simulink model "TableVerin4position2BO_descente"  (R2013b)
settings: Solver=ode15s  StartTime=0.0  StopTime=2  RelTol=1e-3
undefined symbols (not defined in the file): deg, kg, m, mm, N, rad, s, X, Y, Z
libraries: sm_lib x907, fl_lib x25, nesl_utility x19, elec_lib x3, sdl_lib x2
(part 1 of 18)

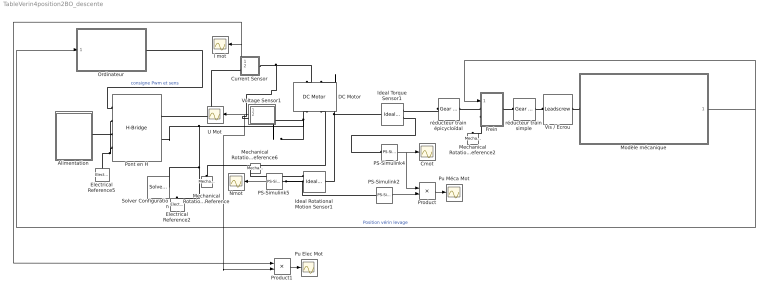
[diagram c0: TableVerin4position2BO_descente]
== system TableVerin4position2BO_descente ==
  Alimentation : Subsystem
  Cmot : Scope
  Current Sensor : Subsystem
  DC Motor : elec_lib/Actuators & Drivers/Rotational Actuators/DC Motor  parameterization=1  Ra=0.53333333 Ohm  La=1600e-6 H  emf_or_torque=2  Kv=0.0637 V/rpm  Ki=0.05555555 N*m/A  T_stall=3e-3*4000/(2*pi*6.25) N*m  w_max=3250 rpm  w_rated=2375 rpm  P_rated=19 W  V_rated=24 V  J=32e-5 kg*m^2  lam_param=2  lam=1e-08 N*m/(rad/s)  i_noload=1.1 A  V_i_noload=24 V  speed0=0 rpm  current_Log=off  voltage_Log=off  power_Log=off  i2r_Log=off  torque_Log=off  speed_Log=off  LocalVarNames=|current|voltage|power|i2r|torque|speed  LocalVarDescs=|Current (A)|Voltage (V)|Power (W)|Electrical losses (W)|Torque (Nm)|Angular speed (rad/s)  LocalVarLogging=[0 0 0 0 0 0]  alpha=0.00393 1/K  Tmeas=25 C  thermal_mass=100 J/K  initial_temperature=25 C
  Electrical Reference2 : fl_lib/Electrical/Electrical Elements/Electrical Reference  i_Log=off  LocalVarNames=|i  LocalVarDescs=|i  LocalVarLogging=[]
  Electrical Reference5 : fl_lib/Electrical/Electrical Elements/Electrical Reference  i_Log=off  LocalVarNames=|i  LocalVarDescs=|i  LocalVarLogging=[]
  Frein : Subsystem
  I mot : Scope
  Ideal Rotational Motion Sensor1 : fl_lib/Mechanical/Mechanical Sensors/Ideal Rotational Motion Sensor  offset=0 deg  w_Log=off  t_Log=off  phi_Log=off  LocalVarNames=|w|t|phi  LocalVarDescs=|w|t|phi  LocalVarLogging=[]
  Ideal Torque Sensor1 : fl_lib/Mechanical/Mechanical Sensors/Ideal Torque Sensor  w_Log=off  t_Log=off  LocalVarNames=|w|t  LocalVarDescs=|w|t  LocalVarLogging=[0 0]
  Mechanical Rotational Reference : fl_lib/Mechanical/Rotational Elements/Mechanical Rotational Reference  t_Log=off  LocalVarNames=|t  LocalVarDescs=|t  LocalVarLogging=[]
  Mechanical Rotational Reference2 : fl_lib/Mechanical/Rotational Elements/Mechanical Rotational Reference  t_Log=off  LocalVarNames=|t  LocalVarDescs=|t  LocalVarLogging=[]
  Mechanical Rotational Reference6 : fl_lib/Mechanical/Rotational Elements/Mechanical Rotational Reference  t_Log=off  LocalVarNames=|t  LocalVarDescs=|t  LocalVarLogging=[]
  Modèle mécanique : Subsystem
  Nmot : Scope
  Ordinateur : Subsystem
  PS-Simulink2 : nesl_utility/PS-Simulink Converter  PhysicalDomain=network_engine_domain  SubClassName=ps_output  LeftPortType=input  RightPortType=output  PseudoPeriodic=off  Frequencies=[]  Unit=rad/s  AffineConversion=off
  PS-Simulink4 : nesl_utility/PS-Simulink Converter  PhysicalDomain=network_engine_domain  SubClassName=ps_output  LeftPortType=input  RightPortType=output  PseudoPeriodic=off  Frequencies=[]  Unit=N*m  AffineConversion=off
  PS-Simulink5 : nesl_utility/PS-Simulink Converter  PhysicalDomain=network_engine_domain  SubClassName=ps_output  LeftPortType=input  RightPortType=output  PseudoPeriodic=off  Frequencies=[]  Unit=rpm  AffineConversion=off
  Pont en H : elec_lib/Actuators & Drivers/Drivers/H-Bridge  Venable=2.5 V  Vmax=5 V  Vreverse=2.5 V  Vbrake=2.5 V  Vm=24 V  pwm_or_av=2  discontinuous=0  freewheeling_mode=1  freewheeling_mode_disc=1  Ron=0.1 Ohm  Don=0.1 Ohm  Rload=10 Ohm  Lload=1e-5 H  F=10 kHz  w_vec=[1, 2] s  i_vec=[1, 2] A  vMatrix=[1, 2; 3, 4] V  iENA_Log=off  iREV_Log=off  iBRK_Log=off  i2_Log=off  v_lag_Log=off  LocalVarNames=|current|voltage|power  LocalVarDescs=|Load current (A)|Load voltage (V)|Load power (W)  LocalVarLogging=[0 0 0]
  Product : Product
  Product1 : Product
  Pu Elec Mot : Scope
  Pu Méca Mot : Scope
  Solver Configuration : nesl_utility/Solver Configuration  PhysicalDomain=network_engine_domain  SubClassName=solver  LeftPortType=input  RightPortType=generic  Accelerate=off  Tones=[]  Harmonics=[]  SimulateNoise=off  Profile=off  UseLocalSampling=off  EnableSwitchedLinearOptims=on  FrequencyDomain=off  UseCCode=off  RelTol=0.001  AbsTol=1e-06  MinStep=1e-09  ToWorkspace=off  DoDC=off  ResidualTolerance=1e-09  UseLocalSolver=off  LocalSolverChoice=NE_BACKWARD_EULER_ADVANCER  LocalSolverSampleTime=0.001  DoFixedCost=off  MaxNonlinIter=3  MaxModeIter=2  LinearAlgebra=Sparse  DelaysMemoryBudget=1024
  U Mot : Scope
  Vis / Ecrou : sdl_lib/Gears/Rotational- Translational/Leadscrew  Lead=0.008 m  helix_type=1  friction_model=2  friction_parameterization=1  lambda=13 deg  alpha=14.5 deg  fr_coeff=0.08  eff_sn=0.75  eff_ns=0.45  mu_visc=0 N*m/(rad/s)  v_thr=0.001 m/s  LocalVarLogging=[]
  Voltage Sensor1 : Subsystem
  réducteur train simple : fl_lib/Mechanical/Mechanisms/Gear Box  ratio=2.98  t_in_Log=off  t_out_Log=off  LocalVarNames=|torque_inp|ang_velocity_inp|power  LocalVarDescs=|Input shaft torque (N*m)|Input shaft angular velocity (rad/s)|Power transmitted by the box (W)  LocalVarLogging=[0 0 0]
  réducteur train épicycloïdal : fl_lib/Mechanical/Mechanisms/Gear Box  ratio=15.44  t_in_Log=off  t_out_Log=off  LocalVarNames=|torque_inp|ang_velocity_inp|power  LocalVarDescs=|Input shaft torque (N*m)|Input shaft angular velocity (rad/s)|Power transmitted by the box (W)  LocalVarLogging=[0 0 0]
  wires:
  Modèle mécanique/1(position) -> Frein/1(freinage), Ordinateur/1(In1)  "Position vérin levage"
  PS-Simulink5/1 -> Nmot/1
  PS-Simulink4/1 -> Product/1, Cmot/1
  Product/1 -> Pu Méca Mot/1
  PS-Simulink2/1 -> Product/2
  Current Sensor/1(i) -> I mot/1, Product1/1
  Product1/1 -> Pu Elec Mot/1
  Voltage Sensor1/2(VuMot2) -> U Mot/1, Product1/2
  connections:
  Vis / Ecrou/LConn1 -- réducteur train simple/RConn1
  Mechanical Rotational Reference/LConn1 -- DC Motor/RConn2
  Frein/LConn2 -- Mechanical Rotational Reference2/LConn1
  Frein/RConn1 -- réducteur train simple/LConn1
  Vis / Ecrou/RConn1 -- Modèle mécanique/LConn1
  DC Motor/RConn1 -- Electrical Reference2/LConn1 -- Solver Configuration/RConn1 -- Pont en H/RConn2 -- Voltage Sensor1/LConn1
  Pont en H/LConn2 -- Electrical Reference5/LConn1 -- Pont en H/LConn4
  Pont en H/LConn1 -- Ordinateur/RConn1  "consigne Pwm et sens"
  Alimentation/RConn1 -- Pont en H/LConn3
  Frein/LConn1 -- réducteur train épicycloïdal/RConn1
  Ideal Rotational Motion Sensor1/LConn1 -- Ideal Torque Sensor1/LConn1 -- DC Motor/LConn2
  Voltage Sensor1/RConn1 -- DC Motor/LConn1 -- Current Sensor/LConn1
  Current Sensor/RConn1 -- Pont en H/RConn1
  Mechanical Rotational Reference6/LConn1 -- Ideal Rotational Motion Sensor1/RConn1
  PS-Simulink5/LConn1 -- PS-Simulink2/LConn1 -- Ideal Rotational Motion Sensor1/RConn2
  Ideal Torque Sensor1/RConn2 -- PS-Simulink4/LConn1
  réducteur train épicycloïdal/LConn1 -- Ideal Torque Sensor1/RConn1

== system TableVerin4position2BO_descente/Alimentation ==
  Constant3 : Constant  Value=5
  Controlled Voltage Source1 : fl_lib/Electrical/Electrical Sources/Controlled Voltage Source  i_Log=off  v_Log=off  LocalVarNames=|i|v  LocalVarDescs=|i|v  LocalVarLogging=[0 0]
  Electrical Reference4 : fl_lib/Electrical/Electrical Elements/Electrical Reference  i_Log=off  LocalVarNames=|i  LocalVarDescs=|i  LocalVarLogging=[]
  Simulink-PS Converter1 : nesl_utility/Simulink-PS Converter  PhysicalDomain=network_engine_domain  SubClassName=ps_input  LeftPortType=input  RightPortType=output  PseudoPeriodic=off  Frequencies=[]  NoiseDistribution=none  NoiseParameters=[]  Unit=V  AffineConversion=off  InputFiltering=off  SimscapeFilterOrder=1  InputFilterTimeConstant=0.001  UdotUserProvided=1
  Conn1 : PMIOPort  Port=1  Side=Right
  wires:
  Constant3/1 -> Simulink-PS Converter1/1
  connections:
  Electrical Reference4/LConn1 -- Controlled Voltage Source1/RConn2
  Simulink-PS Converter1/RConn1 -- Controlled Voltage Source1/RConn1
  Controlled Voltage Source1/LConn1 -- Conn1/RConn1

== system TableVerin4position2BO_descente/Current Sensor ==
  Current Sensor : fl_lib/Electrical/Electrical Sensors/Current Sensor  i1_Log=off  v1_Log=off  LocalVarNames=|i1|v1  LocalVarDescs=|i1|v1  LocalVarLogging=[]
  PS-Simulink Converter 2 : nesl_utility/PS-Simulink Converter  PhysicalDomain=network_engine_domain  SubClassName=ps_output  LeftPortType=input  RightPortType=output  PseudoPeriodic=off  Frequencies=[]  Unit=A  AffineConversion=off
  Volts per unit current : Gain
  + : PMIOPort  Port=1  Side=Right
  - : PMIOPort  Port=2  Side=Left
  i : Outport
  V_i : Outport  Port=2
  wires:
  PS-Simulink Converter 2/1 -> Volts per unit current/1, i/1  "Current (A)"
  Volts per unit current/1 -> V_i/1  "Volts"
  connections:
  +/RConn1 -- Current Sensor/LConn1
  -/RConn1 -- Current Sensor/RConn2
  Current Sensor/RConn1 -- PS-Simulink Converter 2/LConn1

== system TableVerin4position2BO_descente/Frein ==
  note: 240 ou 0
  freinage : Inport
  Constant1 : Constant  Value=0
  Constant2 : Constant  Value=240
  Couple1 : Scope
  Couple2 : Scope
  Ideal Rotational Motion Sensor1 : fl_lib/Mechanical/Mechanical Sensors/Ideal Rotational Motion Sensor  offset=0 deg  w_Log=off  t_Log=off  phi_Log=off  LocalVarNames=|w|t|phi  LocalVarDescs=|w|t|phi  LocalVarLogging=[]
  Ideal Torque Sensor1 : fl_lib/Mechanical/Mechanical Sensors/Ideal Torque Sensor  w_Log=off  t_Log=off  LocalVarNames=|w|t  LocalVarDescs=|w|t  LocalVarLogging=[0 0]
  Ideal Torque Sensor2 : fl_lib/Mechanical/Mechanical Sensors/Ideal Torque Sensor  w_Log=off  t_Log=off  LocalVarNames=|w|t  LocalVarDescs=|w|t  LocalVarLogging=[0 0]
  Loaded-Contact Rotational Friction : sdl_lib/Brakes & Detents/Rotational/Loaded-Contact Rotational Friction  geometry_model=1  r_eff=50 mm  d_o=150 mm  d_i=100 mm  friction_model=1  mu_coulomb=0.2  mu_w_vector=[ 0 0.1 0.2 0.3 0.4 0.5 1 2 5 10 100 1000 ] rad/s  mu_coulomb_vector=[ 0.29 0.28 0.26 0.22 0.21 0.2 0.2 0.19 0.19 0.19 0.19 0.19 ]  mu_interp_method=1  mu_extrap_method=1  mu_static=0.21  w_tol=0.001 rad/s  force_min=0.01 N  mu_visc=0 N*m/(rad/s)  initial_state_locked=0  LocalVarLogging=[]
  Mechanical Rotational Reference6 : fl_lib/Mechanical/Rotational Elements/Mechanical Rotational Reference  t_Log=off  LocalVarNames=|t  LocalVarDescs=|t  LocalVarLogging=[]
  N1 : Scope
  PS-Simulink1 : nesl_utility/PS-Simulink Converter  PhysicalDomain=network_engine_domain  SubClassName=ps_output  LeftPortType=input  RightPortType=output  PseudoPeriodic=off  Frequencies=[]  Unit=N*m  AffineConversion=off
  PS-Simulink4 : nesl_utility/PS-Simulink Converter  PhysicalDomain=network_engine_domain  SubClassName=ps_output  LeftPortType=input  RightPortType=output  PseudoPeriodic=off  Frequencies=[]  Unit=N*m  AffineConversion=off
  PS-Simulink5 : nesl_utility/PS-Simulink Converter  PhysicalDomain=network_engine_domain  SubClassName=ps_output  LeftPortType=input  RightPortType=output  PseudoPeriodic=off  Frequencies=[]  Unit=rpm  AffineConversion=off
  Simulink-PS Converter : nesl_utility/Simulink-PS Converter  PhysicalDomain=network_engine_domain  SubClassName=ps_input  LeftPortType=input  RightPortType=output  PseudoPeriodic=off  Frequencies=[]  NoiseDistribution=none  NoiseParameters=[]  Unit=N  AffineConversion=off  InputFiltering=off  SimscapeFilterOrder=1  InputFilterTimeConstant=0.001  UdotUserProvided=1
  Switch1 : Switch  Criteria=u2 > Threshold  Threshold=-10.172
  force : Scope
  out : PMIOPort  Port=1  Side=Right
  In : PMIOPort  Port=2  Side=Left
  bâti : PMIOPort  Port=3  Side=Left
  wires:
  Switch1/1 -> force/1, Simulink-PS Converter/1
  PS-Simulink5/1 -> N1/1
  PS-Simulink4/1 -> Couple1/1
  Constant1/1 -> Switch1/1
  Constant2/1 -> Switch1/3
  freinage/1 -> Switch1/2
  PS-Simulink1/1 -> Couple2/1
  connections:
  Loaded-Contact Rotational Friction/RConn1 -- Ideal Torque Sensor1/RConn1 -- Ideal Torque Sensor2/LConn1
  PS-Simulink5/LConn1 -- Ideal Rotational Motion Sensor1/RConn2
  Ideal Torque Sensor1/RConn2 -- PS-Simulink4/LConn1
  Loaded-Contact Rotational Friction/LConn1 -- Simulink-PS Converter/RConn1
  Mechanical Rotational Reference6/LConn1 -- Ideal Rotational Motion Sensor1/RConn1
  Ideal Rotational Motion Sensor1/LConn1 -- Ideal Torque Sensor1/LConn1 -- In/RConn1
  bâti/RConn1 -- Loaded-Contact Rotational Friction/LConn2
  Ideal Torque Sensor2/RConn2 -- PS-Simulink1/LConn1
  Ideal Torque Sensor2/RConn1 -- out/RConn1

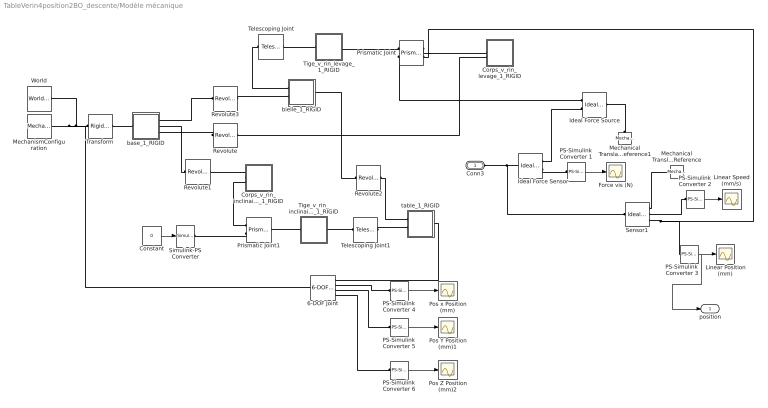
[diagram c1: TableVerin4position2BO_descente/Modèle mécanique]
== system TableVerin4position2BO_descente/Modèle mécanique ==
  6-DOF Joint : sm_lib/Joints/6-DOF Joint  SenseConstraintForceX=off  SenseConstraintForceY=off  SenseConstraintForceZ=off  SenseConstraintTorqueX=off  SenseConstraintTorqueY=off  SenseConstraintTorqueZ=off  ConstraintWrenchDir=FollowerOnBase  ConstraintWrenchFrame=BaseFrame  PxEquilibriumPosition=0  PxEquilibriumPositionUnits=m  PxSpringStiffness=0  PxSpringStiffnessUnits=N/m  PxDampingCoefficient=0  PxDampingCoefficientUnits=N/(m/s)  PxTorqueActuationMode=NoTorque  PxMotionActuationMode=ComputedMotion  PxSensePosition=on  PxSenseVelocity=off  PxSenseAcceleration=off  PxSenseTorqueForce=off  PxPositionTargetValue=0  PxPositionTargetValueUnits=m  PxPositionTargetSpecify=off  PxPositionTargetPriority=High  PxVelocityTargetValue=0  PxVelocityTargetValueUnits=m/s  PxVelocityTargetSpecify=off  PxVelocityTargetPriority=High  PyEquilibriumPosition=0  PyEquilibriumPositionUnits=m  PySpringStiffness=0  PySpringStiffnessUnits=N/m  PyDampingCoefficient=0  PyDampingCoefficientUnits=N/(m/s)  PyTorqueActuationMode=NoTorque  PyMotionActuationMode=ComputedMotion  PySensePosition=on  PySenseVelocity=off  PySenseAcceleration=off  PySenseTorqueForce=off  PyPositionTargetValue=0  PyPositionTargetValueUnits=m  PyPositionTargetSpecify=off  PyPositionTargetPriority=High  PyVelocityTargetValue=0  PyVelocityTargetValueUnits=m/s  PyVelocityTargetSpecify=off  PyVelocityTargetPriority=High  PzEquilibriumPosition=0  PzEquilibriumPositionUnits=m  PzSpringStiffness=0  PzSpringStiffnessUnits=N/m  PzDampingCoefficient=0  PzDampingCoefficientUnits=N/(m/s)  PzTorqueActuationMode=NoTorque  PzMotionActuationMode=ComputedMotion  PzSensePosition=on  PzSenseVelocity=off  PzSenseAcceleration=off  PzSenseTorqueForce=off  PzPositionTargetValue=0  PzPositionTargetValueUnits=m  PzPositionTargetSpecify=off  PzPositionTargetPriority=High  PzVelocityTargetValue=0  PzVelocityTargetValueUnits=m/s  PzVelocityTargetSpecify=off  PzVelocityTargetPriority=High  SphDefPosRotationMethod=None  SphDefPosRotationAngleUnits=deg  SphDefPosRotationStandardAxis=+Z  SphDefPosRotationAngle=0  SphDefPosRotationArbitraryAxis=[0 0 1]  SphDefPosFollAlignAxisA=+X  SphDefPosBaseAlignAxisA=+Y  SphDefPosFollAlignAxisB=+Y  SphDefPosBaseAlignAxisB=+Z  SphEqPosRotationMethod=None  SphEqPosRotationAngleUnits=deg  SphEqPosRotationStandardAxis=+Z  SphEqPosRotationAngle=0  SphEqPosRotationArbitraryAxis=[0 0 1]  SphEqPosFollAlignAxisA=+X  SphEqPosBaseAlignAxisA=+Y  SphEqPosFollAlignAxisB=+Y  SphEqPosBaseAlignAxisB=+Z  SphSpringStiffness=0  SphSpringStiffnessUnits=N*m/deg  SphDampingCoefficient=0  SphDampingCoefficientUnits=N*m/(deg/s)  SphActuateTorqueX=off  SphActuateTorqueY=off  SphActuateTorqueZ=off  SphActuateTorque=off  SphTorqueActuationMode=NoTorque  SphMotionActuationMode=ComputedMotion  SphActuationFrame=BaseFrame  SphSensePosition=off  SphSenseVelocityX=off  SphSenseVelocityY=off  SphSenseVelocityZ=off  SphSenseVelocity=off  SphSenseAccelerationX=off  SphSenseAccelerationY=off  SphSenseAccelerationZ=off  SphSenseAcceleration=off  SphSenseTorqueX=off  SphSenseTorqueY=off  SphSenseTorqueZ=off  SphSenseTorqueForce=off  SphSensingFrame=BaseFrame  SphPositionTargetRotationMethod=None  SphPositionTargetRotationAngleUnits=deg  SphPositionTargetRotationStandardAxis=+Z  SphPositionTargetRotationAngle=0  SphPositionTargetRotationArbitraryAxis=[0 0 1]  SphPositionTargetFollAlignAxisA=+X  SphPositionTargetBaseAlignAxisA=+Y  SphPositionTargetFollAlignAxisB=+Y  SphPositionTargetBaseAlignAxisB=+Z  SphPositionTargetSpecify=off  SphPositionTargetPriority=High  SphVelocityTargetValue=[0 0 0]  SphVelocityTargetValueUnits=deg/s  SphVelocityTargetSpecify=off  SphVelocityTargetPriority=High  SphVelocityTargetInFollowerFrame=on  BlockFunction=simmechanics.library.joints.sixdof_joint
  Constant : Constant  Value=0
  Corps_v_rin_inclinaison_1_RIGID : Subsystem
  Corps_v_rin_levage_1_RIGID : Subsystem
  Force vis (N) : Scope
  Ideal Force Sensor : fl_lib/Mechanical/Mechanical Sensors/Ideal Force Sensor  v_Log=off  f_Log=off  LocalVarNames=|v|f  LocalVarDescs=|v|f  LocalVarLogging=[0 0]
  Ideal Force Source : fl_lib/Mechanical/Mechanical Sources/Ideal Force Source  v_Log=off  f_Log=off  LocalVarNames=|v|f  LocalVarDescs=|v|f  LocalVarLogging=[0 0]
  Linear Position (mm) : Scope
  Linear Speed (mm/s) : Scope
  Mechanical Translational Reference : fl_lib/Mechanical/Translational Elements/Mechanical Translational Reference  f_Log=off  LocalVarNames=|f  LocalVarDescs=|f  LocalVarLogging=[]
  Mechanical Translational Reference1 : fl_lib/Mechanical/Translational Elements/Mechanical Translational Reference  f_Log=off  LocalVarNames=|f  LocalVarDescs=|f  LocalVarLogging=[]
  MechanismConfiguration : sm_lib/Utilities/Mechanism Configuration  GravityVector=[0 0 -9.81]  GravityUnits=m/s^2  AllowGravitySignal=off  LinearizationDelta=0.001  BlockFunction=simmechanics.library.utilities.mechanism_configuration
  PS-Simulink Converter 1 : nesl_utility/PS-Simulink Converter  PhysicalDomain=network_engine_domain  SubClassName=ps_output  LeftPortType=input  RightPortType=output  PseudoPeriodic=off  Frequencies=[]  Unit=N  AffineConversion=off
  PS-Simulink Converter 2 : nesl_utility/PS-Simulink Converter  PhysicalDomain=network_engine_domain  SubClassName=ps_output  LeftPortType=input  RightPortType=output  PseudoPeriodic=off  Frequencies=[]  Unit=mm/s  AffineConversion=off
  PS-Simulink Converter {3..6} (4 alike) : nesl_utility/PS-Simulink Converter  PhysicalDomain=network_engine_domain  SubClassName=ps_output  LeftPortType=input  RightPortType=output  PseudoPeriodic=off  Frequencies=[]  Unit=mm  AffineConversion=off
  Pos Y Position (mm)1 : Scope
  Pos Z Position (mm)2 : Scope
  Pos x Position (mm) : Scope
  Prismatic Joint : sm_lib/Joints/Prismatic Joint  SenseConstraintForceX=off  SenseConstraintForceY=off  SenseConstraintForceZ=off  SenseConstraintTorqueX=off  SenseConstraintTorqueY=off  SenseConstraintTorqueZ=off  ConstraintWrenchDir=FollowerOnBase  ConstraintWrenchFrame=BaseFrame  EquilibriumPosition=0  EquilibriumPositionUnits=m  SpringStiffness=0  SpringStiffnessUnits=N/m  DampingCoefficient=0  DampingCoefficientUnits=N/(m/s)  TorqueActuationMode=ComputedTorque  MotionActuationMode=InputMotion  SensePosition=off  SenseVelocity=off  SenseAcceleration=off  SenseTorqueForce=on  PositionTargetValue=0  PositionTargetValueUnits=m  PositionTargetSpecify=off  PositionTargetPriority=High  VelocityTargetValue=0  VelocityTargetValueUnits=m/s  VelocityTargetSpecify=off  VelocityTargetPriority=High  BlockFunction=simmechanics.library.joints.prismatic_joint
  Prismatic Joint1 : sm_lib/Joints/Prismatic Joint  SenseConstraintForceX=off  SenseConstraintForceY=off  SenseConstraintForceZ=off  SenseConstraintTorqueX=off  SenseConstraintTorqueY=off  SenseConstraintTorqueZ=off  ConstraintWrenchDir=FollowerOnBase  ConstraintWrenchFrame=BaseFrame  EquilibriumPosition=0  EquilibriumPositionUnits=m  SpringStiffness=0  SpringStiffnessUnits=N/m  DampingCoefficient=0  DampingCoefficientUnits=N/(m/s)  TorqueActuationMode=ComputedTorque  MotionActuationMode=InputMotion  SensePosition=off  SenseVelocity=off  SenseAcceleration=off  SenseTorqueForce=off  PositionTargetValue=0  PositionTargetValueUnits=m  PositionTargetSpecify=off  PositionTargetPriority=High  VelocityTargetValue=0  VelocityTargetValueUnits=m/s  VelocityTargetSpecify=off  VelocityTargetPriority=High  BlockFunction=simmechanics.library.joints.prismatic_joint
  Revolute : sm_lib/Joints/Revolute Joint  SenseConstraintForceX=off  SenseConstraintForceY=off  SenseConstraintForceZ=off  SenseConstraintTorqueX=off  SenseConstraintTorqueY=off  SenseConstraintTorqueZ=off  ConstraintWrenchDir=FollowerOnBase  ConstraintWrenchFrame=BaseFrame  EquilibriumPosition=0  EquilibriumPositionUnits=rad  SpringStiffness=0  SpringStiffnessUnits=m*N/rad  DampingCoefficient=0  DampingCoefficientUnits=m*s*N/rad  TorqueActuationMode=NoTorque  MotionActuationMode=ComputedMotion  SensePosition=off  SenseVelocity=off  SenseAcceleration=off  SenseTorqueForce=off  PositionTargetValue=-19.448954484523508  PositionTargetValueUnits=deg  PositionTargetSpecify=on  PositionTargetPriority=Low  VelocityTargetValue=0  VelocityTargetValueUnits=deg/s  VelocityTargetSpecify=off  VelocityTargetPriority=High  BlockFunction=simmechanics.library.joints.revolute_joint
  Revolute1 : sm_lib/Joints/Revolute Joint  SenseConstraintForceX=off  SenseConstraintForceY=off  SenseConstraintForceZ=off  SenseConstraintTorqueX=off  SenseConstraintTorqueY=off  SenseConstraintTorqueZ=off  ConstraintWrenchDir=FollowerOnBase  ConstraintWrenchFrame=BaseFrame  EquilibriumPosition=0  EquilibriumPositionUnits=rad  SpringStiffness=0  SpringStiffnessUnits=m*N/rad  DampingCoefficient=0  DampingCoefficientUnits=m*s*N/rad  TorqueActuationMode=NoTorque  MotionActuationMode=ComputedMotion  SensePosition=off  SenseVelocity=off  SenseAcceleration=off  SenseTorqueForce=off  PositionTargetValue=-0.69151960924487288  PositionTargetValueUnits=deg  PositionTargetSpecify=on  PositionTargetPriority=Low  VelocityTargetValue=0  VelocityTargetValueUnits=deg/s  VelocityTargetSpecify=off  VelocityTargetPriority=High  BlockFunction=simmechanics.library.joints.revolute_joint
  Revolute2 : sm_lib/Joints/Revolute Joint  SenseConstraintForceX=off  SenseConstraintForceY=off  SenseConstraintForceZ=off  SenseConstraintTorqueX=off  SenseConstraintTorqueY=off  SenseConstraintTorqueZ=off  ConstraintWrenchDir=FollowerOnBase  ConstraintWrenchFrame=BaseFrame  EquilibriumPosition=0  EquilibriumPositionUnits=rad  SpringStiffness=0  SpringStiffnessUnits=m*N/rad  DampingCoefficient=0  DampingCoefficientUnits=m*s*N/rad  TorqueActuationMode=NoTorque  MotionActuationMode=ComputedMotion  SensePosition=off  SenseVelocity=off  SenseAcceleration=off  SenseTorqueForce=off  PositionTargetValue=37.808774161373094  PositionTargetValueUnits=deg  PositionTargetSpecify=on  PositionTargetPriority=Low  VelocityTargetValue=0  VelocityTargetValueUnits=deg/s  VelocityTargetSpecify=off  VelocityTargetPriority=High  BlockFunction=simmechanics.library.joints.revolute_joint
  Revolute3 : sm_lib/Joints/Revolute Joint  SenseConstraintForceX=off  SenseConstraintForceY=off  SenseConstraintForceZ=off  SenseConstraintTorqueX=off  SenseConstraintTorqueY=off  SenseConstraintTorqueZ=off  ConstraintWrenchDir=FollowerOnBase  ConstraintWrenchFrame=BaseFrame  EquilibriumPosition=0  EquilibriumPositionUnits=rad  SpringStiffness=0  SpringStiffnessUnits=m*N/rad  DampingCoefficient=0  DampingCoefficientUnits=m*s*N/rad  TorqueActuationMode=NoTorque  MotionActuationMode=ComputedMotion  SensePosition=off  SenseVelocity=off  SenseAcceleration=off  SenseTorqueForce=off  PositionTargetValue=-37.808774161373101  PositionTargetValueUnits=deg  PositionTargetSpecify=on  PositionTargetPriority=Low  VelocityTargetValue=0  VelocityTargetValueUnits=deg/s  VelocityTargetSpecify=off  VelocityTargetPriority=High  BlockFunction=simmechanics.library.joints.revolute_joint
  Sensor1 : fl_lib/Mechanical/Mechanical Sensors/Ideal Translational Motion Sensor  offset=0 m  v_Log=off  f_Log=off  x_Log=off  LocalVarNames=|v|f|x  LocalVarDescs=|v|f|x  LocalVarLogging=[]
  Simulink-PS Converter : nesl_utility/Simulink-PS Converter  PhysicalDomain=network_engine_domain  SubClassName=ps_input  LeftPortType=input  RightPortType=output  PseudoPeriodic=off  Frequencies=[]  NoiseDistribution=none  NoiseParameters=[]  Unit=m  AffineConversion=off  InputFiltering=off  SimscapeFilterOrder=1  InputFilterTimeConstant=0.001  UdotUserProvided=1
  Telescoping Joint : sm_lib/Joints/Telescoping Joint  SenseConstraintForceX=off  SenseConstraintForceY=off  SenseConstraintForceZ=off  SenseConstraintTorqueX=off  SenseConstraintTorqueY=off  SenseConstraintTorqueZ=off  ConstraintWrenchDir=FollowerOnBase  ConstraintWrenchFrame=BaseFrame  SphDefPosRotationMethod=None  SphDefPosRotationAngleUnits=deg  SphDefPosRotationStandardAxis=+Z  SphDefPosRotationAngle=0  SphDefPosRotationArbitraryAxis=[0 0 1]  SphDefPosFollAlignAxisA=+X  SphDefPosBaseAlignAxisA=+Y  SphDefPosFollAlignAxisB=+Y  SphDefPosBaseAlignAxisB=+Z  SphEqPosRotationMethod=None  SphEqPosRotationAngleUnits=deg  SphEqPosRotationStandardAxis=+Z  SphEqPosRotationAngle=0  SphEqPosRotationArbitraryAxis=[0 0 1]  SphEqPosFollAlignAxisA=+X  SphEqPosBaseAlignAxisA=+Y  SphEqPosFollAlignAxisB=+Y  SphEqPosBaseAlignAxisB=+Z  SphSpringStiffness=0  SphSpringStiffnessUnits=N*m/deg  SphDampingCoefficient=0  SphDampingCoefficientUnits=N*m/(deg/s)  SphActuateTorqueX=off  SphActuateTorqueY=off  SphActuateTorqueZ=off  SphActuateTorque=off  SphTorqueActuationMode=NoTorque  SphMotionActuationMode=ComputedMotion  SphActuationFrame=BaseFrame  SphSensePosition=off  SphSenseVelocityX=off  SphSenseVelocityY=off  SphSenseVelocityZ=off  SphSenseVelocity=off  SphSenseAccelerationX=off  SphSenseAccelerationY=off  SphSenseAccelerationZ=off  SphSenseAcceleration=off  SphSenseTorqueX=off  SphSenseTorqueY=off  SphSenseTorqueZ=off  SphSenseTorqueForce=off  SphSensingFrame=BaseFrame  SphPositionTargetRotationMethod=None  SphPositionTargetRotationAngleUnits=deg  SphPositionTargetRotationStandardAxis=+Z  SphPositionTargetRotationAngle=0  SphPositionTargetRotationArbitraryAxis=[0 0 1]  SphPositionTargetFollAlignAxisA=+X  SphPositionTargetBaseAlignAxisA=+Y  SphPositionTargetFollAlignAxisB=+Y  SphPositionTargetBaseAlignAxisB=+Z  SphPositionTargetSpecify=off  SphPositionTargetPriority=High  SphVelocityTargetValue=[0 0 0]  SphVelocityTargetValueUnits=deg/s  SphVelocityTargetSpecify=off  SphVelocityTargetPriority=High  SphVelocityTargetInFollowerFrame=on  PzEquilibriumPosition=0  PzEquilibriumPositionUnits=m  PzSpringStiffness=0  PzSpringStiffnessUnits=N/m  PzDampingCoefficient=0  PzDampingCoefficientUnits=N/(m/s)  PzTorqueActuationMode=NoTorque  PzMotionActuationMode=ComputedMotion  PzSensePosition=off  PzSenseVelocity=off  PzSenseAcceleration=off  PzSenseTorqueForce=off  PzPositionTargetValue=0  PzPositionTargetValueUnits=m  PzPositionTargetSpecify=off  PzPositionTargetPriority=High  PzVelocityTargetValue=0  PzVelocityTargetValueUnits=m/s  PzVelocityTargetSpecify=off  PzVelocityTargetPriority=High  BlockFunction=simmechanics.library.joints.telescoping_joint
  Telescoping Joint1 : sm_lib/Joints/Telescoping Joint  SenseConstraintForceX=off  SenseConstraintForceY=off  SenseConstraintForceZ=off  SenseConstraintTorqueX=off  SenseConstraintTorqueY=off  SenseConstraintTorqueZ=off  ConstraintWrenchDir=FollowerOnBase  ConstraintWrenchFrame=BaseFrame  SphDefPosRotationMethod=None  SphDefPosRotationAngleUnits=deg  SphDefPosRotationStandardAxis=+Z  SphDefPosRotationAngle=0  SphDefPosRotationArbitraryAxis=[0 0 1]  SphDefPosFollAlignAxisA=+X  SphDefPosBaseAlignAxisA=+Y  SphDefPosFollAlignAxisB=+Y  SphDefPosBaseAlignAxisB=+Z  SphEqPosRotationMethod=None  SphEqPosRotationAngleUnits=deg  SphEqPosRotationStandardAxis=+Z  SphEqPosRotationAngle=0  SphEqPosRotationArbitraryAxis=[0 0 1]  SphEqPosFollAlignAxisA=+X  SphEqPosBaseAlignAxisA=+Y  SphEqPosFollAlignAxisB=+Y  SphEqPosBaseAlignAxisB=+Z  SphSpringStiffness=0  SphSpringStiffnessUnits=N*m/deg  SphDampingCoefficient=0  SphDampingCoefficientUnits=N*m/(deg/s)  SphActuateTorqueX=off  SphActuateTorqueY=off  SphActuateTorqueZ=off  SphActuateTorque=off  SphTorqueActuationMode=NoTorque  SphMotionActuationMode=ComputedMotion  SphActuationFrame=BaseFrame  SphSensePosition=off  SphSenseVelocityX=off  SphSenseVelocityY=off  SphSenseVelocityZ=off  SphSenseVelocity=off  SphSenseAccelerationX=off  SphSenseAccelerationY=off  SphSenseAccelerationZ=off  SphSenseAcceleration=off  SphSenseTorqueX=off  SphSenseTorqueY=off  SphSenseTorqueZ=off  SphSenseTorqueForce=off  SphSensingFrame=BaseFrame  SphPositionTargetRotationMethod=None  SphPositionTargetRotationAngleUnits=deg  SphPositionTargetRotationStandardAxis=+Z  SphPositionTargetRotationAngle=0  SphPositionTargetRotationArbitraryAxis=[0 0 1]  SphPositionTargetFollAlignAxisA=+X  SphPositionTargetBaseAlignAxisA=+Y  SphPositionTargetFollAlignAxisB=+Y  SphPositionTargetBaseAlignAxisB=+Z  SphPositionTargetSpecify=off  SphPositionTargetPriority=High  SphVelocityTargetValue=[0 0 0]  SphVelocityTargetValueUnits=deg/s  SphVelocityTargetSpecify=off  SphVelocityTargetPriority=High  SphVelocityTargetInFollowerFrame=on  PzEquilibriumPosition=0  PzEquilibriumPositionUnits=m  PzSpringStiffness=0  PzSpringStiffnessUnits=N/m  PzDampingCoefficient=0  PzDampingCoefficientUnits=N/(m/s)  PzTorqueActuationMode=NoTorque  PzMotionActuationMode=ComputedMotion  PzSensePosition=off  PzSenseVelocity=off  PzSenseAcceleration=off  PzSenseTorqueForce=off  PzPositionTargetValue=0  PzPositionTargetValueUnits=m  PzPositionTargetSpecify=off  PzPositionTargetPriority=High  PzVelocityTargetValue=0  PzVelocityTargetValueUnits=m/s  PzVelocityTargetSpecify=off  PzVelocityTargetPriority=High  BlockFunction=simmechanics.library.joints.telescoping_joint
  Tige_v_rin_inclinaison_1_RIGID : Subsystem
  Tige_v_rin_levage_1_RIGID : Subsystem
  Transform : sm_lib/Frames and Transforms/Rigid Transform  TranslationMethod=Cartesian  TranslationLengthUnit=mm  TranslationStandardAxis=+Z  TranslationStandardOffset=0  TranslationCartesianOffset=[-44.940899999999999 -2.2279000000000001e-11 85]  TranslationROffset=0  TranslationROffsetUnits=m  TranslationZOffset=0  TranslationZOffsetUnits=m  TranslationThetaOffset=0  TranslationThetaOffsetUnits=deg  RotationMethod=None  RotationAngleUnits=deg  RotationStandardAxis=+Z  RotationAngle=0  RotationArbitraryAxis=[0 0 1]  FollAlignAxisA=+X  BaseAlignAxisA=+Y  FollAlignAxisB=+Y  BaseAlignAxisB=+Z  BlockFunction=simmechanics.library.frames_transforms.rigid_transform
  World : sm_lib/Frames and Transforms/World Frame  BlockFunction=simmechanics.library.frames_transforms.world_frame
  base_1_RIGID : Subsystem
  bielle_1_RIGID : Subsystem
  table_1_RIGID : Subsystem
  Conn3 : PMIOPort  Port=1  Side=Left
  position : Outport
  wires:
  Constant/1 -> Simulink-PS Converter/1
  PS-Simulink Converter 3/1 -> position/1, Linear Position (mm)/1
  PS-Simulink Converter 2/1 -> Linear Speed (mm/s)/1
  PS-Simulink Converter 1/1 -> Force vis (N)/1
  PS-Simulink Converter 4/1 -> Pos x Position (mm)/1
  PS-Simulink Converter 5/1 -> Pos Y Position (mm)1/1
  PS-Simulink Converter 6/1 -> Pos Z Position (mm)2/1
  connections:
  Revolute/LConn1 -- base_1_RIGID/RConn3
  MechanismConfiguration/RConn1 -- World/RConn1 -- 6-DOF Joint/LConn1 -- Transform/LConn1
  Revolute2/RConn1 -- table_1_RIGID/LConn1
  Revolute2/LConn1 -- bielle_1_RIGID/RConn1
  Corps_v_rin_levage_1_RIGID/LConn2 -- Revolute/RConn1
  Prismatic Joint1/RConn1 -- Tige_v_rin_inclinaison_1_RIGID/RConn1
  Transform/RConn1 -- base_1_RIGID/LConn1
  Revolute3/RConn1 -- bielle_1_RIGID/LConn2
  Revolute3/LConn1 -- base_1_RIGID/RConn1
  Prismatic Joint1/LConn1 -- Corps_v_rin_inclinaison_1_RIGID/LConn2
  bielle_1_RIGID/LConn1 -- Telescoping Joint/LConn1
  Telescoping Joint/RConn1 -- Tige_v_rin_levage_1_RIGID/LConn1
  Sensor1/LConn1 -- Ideal Force Sensor/LConn1 -- Conn3/RConn1
  Telescoping Joint1/RConn1 -- table_1_RIGID/LConn2
  Tige_v_rin_inclinaison_1_RIGID/LConn1 -- Telescoping Joint1/LConn1
  Ideal Force Source/RConn1 -- Prismatic Joint/RConn2
  Prismatic Joint/LConn1 -- Corps_v_rin_levage_1_RIGID/LConn1
  Corps_v_rin_inclinaison_1_RIGID/LConn1 -- Revolute1/RConn1
  Mechanical Translational Reference1/LConn1 -- Ideal Force Source/LConn1
  Tige_v_rin_levage_1_RIGID/RConn1 -- Prismatic Joint/RConn1
  Revolute1/LConn1 -- base_1_RIGID/RConn2
  Prismatic Joint1/LConn2 -- Simulink-PS Converter/RConn1
  Prismatic Joint/LConn2 -- PS-Simulink Converter 3/LConn1 -- Sensor1/RConn3
  Sensor1/RConn1 -- Mechanical Translational Reference/LConn1
  PS-Simulink Converter 2/LConn1 -- Sensor1/RConn2
  Ideal Force Sensor/RConn2 -- PS-Simulink Converter 1/LConn1
  Ideal Force Sensor/RConn1 -- Ideal Force Source/RConn2
  6-DOF Joint/RConn1 -- table_1_RIGID/RConn1
  6-DOF Joint/RConn2 -- PS-Simulink Converter 4/LConn1
  PS-Simulink Converter 5/LConn1 -- 6-DOF Joint/RConn3
  PS-Simulink Converter 6/LConn1 -- 6-DOF Joint/RConn4

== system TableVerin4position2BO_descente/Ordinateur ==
  In1 : Inport
  5volts/4000rpm : Gain  Gain=5/4000
  Constant4 : Constant  Value=0
  Constant5 : Constant  Value=4000
  Controlled PWM Voltage : elec_lib/Actuators & Drivers/Drivers/Controlled PWM Voltage  F=10000 Hz  TD=0 s  pulse_width_offset=0 s  Vmin=0 V  Vmax=5 V  Vm=5 V  pwm_or_av=2  event_type=1  sample_time=1e-6 s  LocalVarNames=|current|voltage|power  LocalVarDescs=|Load current (A)|Load voltage (V)|Load power (W)  LocalVarLogging=[0 0 0]
  Controlled Voltage Source : fl_lib/Electrical/Electrical Sources/Controlled Voltage Source  i_Log=off  v_Log=off  LocalVarNames=|i|v  LocalVarDescs=|i|v  LocalVarLogging=[0 0]
  Electrical Reference1 : fl_lib/Electrical/Electrical Elements/Electrical Reference  i_Log=off  LocalVarNames=|i  LocalVarDescs=|i  LocalVarLogging=[]
  Electrical Reference3 : fl_lib/Electrical/Electrical Elements/Electrical Reference  i_Log=off  LocalVarNames=|i  LocalVarDescs=|i  LocalVarLogging=[]
  Simulink-PS Converter : nesl_utility/Simulink-PS Converter  PhysicalDomain=network_engine_domain  SubClassName=ps_input  LeftPortType=input  RightPortType=output  PseudoPeriodic=off  Frequencies=[]  NoiseDistribution=none  NoiseParameters=[]  Unit=V  AffineConversion=off  InputFiltering=off  SimscapeFilterOrder=1  InputFilterTimeConstant=0.001  UdotUserProvided=1
  Switch : Switch  Criteria=u2 > Threshold  Threshold=-10.172
  consVitesse : Scope
  retour Position : Scope
  Conn1 : PMIOPort  Port=1  Side=Right
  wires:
  Constant5/1 -> Switch/1
  Switch/1 -> 5volts/4000rpm/1, consVitesse/1
  In1/1 -> retour Position/1, Switch/2
  5volts/4000rpm/1 -> Simulink-PS Converter/1
  Constant4/1 -> Switch/3
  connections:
  Controlled Voltage Source/LConn1 -- Controlled PWM Voltage/LConn1
  Conn1/RConn1 -- Controlled PWM Voltage/RConn1
  Controlled PWM Voltage/RConn2 -- Controlled PWM Voltage/LConn2 -- Electrical Reference1/LConn1
  Simulink-PS Converter/RConn1 -- Controlled Voltage Source/RConn1
  Electrical Reference3/LConn1 -- Controlled Voltage Source/RConn2

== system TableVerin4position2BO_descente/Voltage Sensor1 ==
  PS-Simulink Converter 2 : nesl_utility/PS-Simulink Converter  PhysicalDomain=network_engine_domain  SubClassName=ps_output  LeftPortType=input  RightPortType=output  PseudoPeriodic=off  Frequencies=[]  Unit=V  AffineConversion=off
  Voltage Sensor : fl_lib/Electrical/Electrical Sensors/Voltage Sensor  i1_Log=off  v1_Log=off  LocalVarNames=|i1|v1  LocalVarDescs=|i1|v1  LocalVarLogging=[0 0]
  + : PMIOPort  Port=1  Side=Right
  - : PMIOPort  Port=2  Side=Left
  uMot : Outport
  VuMot2 : Outport  Port=2
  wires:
  PS-Simulink Converter 2/1 -> VuMot2/1, uMot/1  "Tension (V)"
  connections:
  Voltage Sensor/LConn1 -- +/RConn1
  -/RConn1 -- Voltage Sensor/RConn2
  Voltage Sensor/RConn1 -- PS-Simulink Converter 2/LConn1

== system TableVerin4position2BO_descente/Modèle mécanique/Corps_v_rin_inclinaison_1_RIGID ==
  ReferenceFrame : sm_lib/Frames and Transforms/Reference Frame  BlockFunction=simmechanics.library.frames_transforms.reference_frame
  Transform : sm_lib/Frames and Transforms/Rigid Transform  TranslationMethod=Cartesian  TranslationLengthUnit=mm  TranslationStandardAxis=+Z  TranslationStandardOffset=0  TranslationCartesianOffset=[581.58897838011512 -79.972299999999905 18.779086684198781]  TranslationROffset=0  TranslationROffsetUnits=m  TranslationZOffset=0  TranslationZOffsetUnits=m  TranslationThetaOffset=0  TranslationThetaOffsetUnits=deg  RotationMethod=ArbitraryAxis  RotationAngleUnits=rad  RotationStandardAxis=+Z  RotationAngle=2.0943951023931957  RotationArbitraryAxis=[0.57735026918962573 0.57735026918962584 0.57735026918962573]  FollAlignAxisA=+X  BaseAlignAxisA=+Y  FollAlignAxisB=+Y  BaseAlignAxisB=+Z  BlockFunction=simmechanics.library.frames_transforms.rigid_transform
  Transform1 : sm_lib/Frames and Transforms/Rigid Transform  TranslationMethod=Cartesian  TranslationLengthUnit=mm  TranslationStandardAxis=+Z  TranslationStandardOffset=0  TranslationCartesianOffset=[16.943688345754151 -124.27970000002227 18.779161135203918]  TranslationROffset=0  TranslationROffsetUnits=m  TranslationZOffset=0  TranslationZOffsetUnits=m  TranslationThetaOffset=0  TranslationThetaOffsetUnits=deg  RotationMethod=ArbitraryAxis  RotationAngleUnits=rad  RotationStandardAxis=+Z  RotationAngle=2.0943951023931957  RotationArbitraryAxis=[0.57735026918962584 -0.57735026918962551 0.57735026918962595]  FollAlignAxisA=+X  BaseAlignAxisA=+Y  FollAlignAxisB=+Y  BaseAlignAxisB=+Z  BlockFunction=simmechanics.library.frames_transforms.rigid_transform
  Transform2 : sm_lib/Frames and Transforms/Rigid Transform  TranslationMethod=Cartesian  TranslationLengthUnit=mm  TranslationStandardAxis=+Z  TranslationStandardOffset=0  TranslationCartesianOffset=[223.357 -79.97229999999999 92.199100000000001]  TranslationROffset=0  TranslationROffsetUnits=m  TranslationZOffset=0  TranslationZOffsetUnits=m  TranslationThetaOffset=0  TranslationThetaOffsetUnits=deg  RotationMethod=ArbitraryAxis  RotationAngleUnits=rad  RotationStandardAxis=+Z  RotationAngle=3.1415926535897931  RotationArbitraryAxis=[-0.70710678118654746 -5.2401915786782071e-17 -0.70710678118654757]  FollAlignAxisA=+X  BaseAlignAxisA=+Y  FollAlignAxisB=+Y  BaseAlignAxisB=+Z  BlockFunction=simmechanics.library.frames_transforms.rigid_transform
  Transform3 : sm_lib/Frames and Transforms/Rigid Transform  TranslationMethod=Cartesian  TranslationLengthUnit=mm  TranslationStandardAxis=+Z  TranslationStandardOffset=0  TranslationCartesianOffset=[61.256599999999999 -79.97229999999999 18.7791]  TranslationROffset=0  TranslationROffsetUnits=m  TranslationZOffset=0  TranslationZOffsetUnits=m  TranslationThetaOffset=0  TranslationThetaOffsetUnits=deg  RotationMethod=ArbitraryAxis  RotationAngleUnits=rad  RotationStandardAxis=+Z  RotationAngle=1.6178481128137681  RotationArbitraryAxis=[0.21194708467810194 -0.21194708467810194 0.95402141830930975]  FollAlignAxisA=+X  BaseAlignAxisA=+Y  FollAlignAxisB=+Y  BaseAlignAxisB=+Z  BlockFunction=simmechanics.library.frames_transforms.rigid_transform
  Transform4 : sm_lib/Frames and Transforms/Rigid Transform  TranslationMethod=Cartesian  TranslationLengthUnit=mm  TranslationStandardAxis=+Z  TranslationStandardOffset=0  TranslationCartesianOffset=[16.944099999999999 -79.97229999999999 18.7791]  TranslationROffset=0  TranslationROffsetUnits=m  TranslationZOffset=0  TranslationZOffsetUnits=m  TranslationThetaOffset=0  TranslationThetaOffsetUnits=deg  RotationMethod=None  RotationAngleUnits=deg  RotationStandardAxis=+Z  RotationAngle=0  RotationArbitraryAxis=[0 0 1]  FollAlignAxisA=+X  BaseAlignAxisA=+Y  FollAlignAxisB=+Y  BaseAlignAxisB=+Z  BlockFunction=simmechanics.library.frames_transforms.rigid_transform
  Transform5 : sm_lib/Frames and Transforms/Rigid Transform  TranslationMethod=Cartesian  TranslationLengthUnit=mm  TranslationStandardAxis=+Z  TranslationStandardOffset=0  TranslationCartesianOffset=[117.25700000000001 -79.97229999999999 18.7791]  TranslationROffset=0  TranslationROffsetUnits=m  TranslationZOffset=0  TranslationZOffsetUnits=m  TranslationThetaOffset=0  TranslationThetaOffsetUnits=deg  RotationMethod=ArbitraryAxis  RotationAngleUnits=rad  RotationStandardAxis=+Z  RotationAngle=3.1415926535897931  RotationArbitraryAxis=[0 0.97311979050629582 0.2302995295804641]  FollAlignAxisA=+X  BaseAlignAxisA=+Y  FollAlignAxisB=+Y  BaseAlignAxisB=+Z  BlockFunction=simmechanics.library.frames_transforms.rigid_transform
  x15060_Ecrou_24_Ecrou_Hm_M16_1_RIGID : Subsystem
  x15060_M_01073_Interface_ar_verin_AA_DEFAULT_1_RIGID : Subsystem
  x15060_NLM_Embout_a_rotule_M16_Pas_a_droite_27627_16_1_RIGID : Subsystem
  x15060_Verin_LA36_Course_100_mm_1_RIGID : Subsystem
  F1 : PMIOPort  Port=1  Side=Left
  F : PMIOPort  Port=2  Side=Left
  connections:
  Transform/LConn1 -- ReferenceFrame/RConn1 -- Transform1/LConn1 -- Transform2/LConn1 -- Transform3/LConn1 -- Transform4/LConn1 -- Transform5/LConn1
  Transform/RConn1 -- F/RConn1
  Transform1/RConn1 -- F1/RConn1
  Transform2/RConn1 -- x15060_Verin_LA36_Course_100_mm_1_RIGID/LConn1
  Transform3/RConn1 -- x15060_Ecrou_24_Ecrou_Hm_M16_1_RIGID/LConn1
  Transform4/RConn1 -- x15060_NLM_Embout_a_rotule_M16_Pas_a_droite_27627_16_1_RIGID/LConn1
  Transform5/RConn1 -- x15060_M_01073_Interface_ar_verin_AA_DEFAULT_1_RIGID/LConn1

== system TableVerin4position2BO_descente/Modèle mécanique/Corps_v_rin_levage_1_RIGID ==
  ReferenceFrame : sm_lib/Frames and Transforms/Reference Frame  BlockFunction=simmechanics.library.frames_transforms.reference_frame
  Transform : sm_lib/Frames and Transforms/Rigid Transform  TranslationMethod=Cartesian  TranslationLengthUnit=mm  TranslationStandardAxis=+Z  TranslationStandardOffset=0  TranslationCartesianOffset=[16.948520761169686 32.492699999977624 18.777580013894262]  TranslationROffset=0  TranslationROffsetUnits=m  TranslationZOffset=0  TranslationZOffsetUnits=m  TranslationThetaOffset=0  TranslationThetaOffsetUnits=deg  RotationMethod=ArbitraryAxis  RotationAngleUnits=rad  RotationStandardAxis=+Z  RotationAngle=2.0943951023931935  RotationArbitraryAxis=[-0.57735026918962506 -0.57735026918962595 -0.5773502691896264]  FollAlignAxisA=+X  BaseAlignAxisA=+Y  FollAlignAxisB=+Y  BaseAlignAxisB=+Z  BlockFunction=simmechanics.library.frames_transforms.rigid_transform
  Transform1 : sm_lib/Frames and Transforms/Rigid Transform  TranslationMethod=Cartesian  TranslationLengthUnit=mm  TranslationStandardAxis=+Z  TranslationStandardOffset=0  TranslationCartesianOffset=[449.09427593857532 -79.972300000000033 18.776101630550443]  TranslationROffset=0  TranslationROffsetUnits=m  TranslationZOffset=0  TranslationZOffsetUnits=m  TranslationThetaOffset=0  TranslationThetaOffsetUnits=deg  RotationMethod=ArbitraryAxis  RotationAngleUnits=rad  RotationStandardAxis=+Z  RotationAngle=2.0943951023931953  RotationArbitraryAxis=[0.57735026918962551 0.57735026918962562 0.57735026918962606]  FollAlignAxisA=+X  BaseAlignAxisA=+Y  FollAlignAxisB=+Y  BaseAlignAxisB=+Z  BlockFunction=simmechanics.library.frames_transforms.rigid_transform
  Transform2 : sm_lib/Frames and Transforms/Rigid Transform  TranslationMethod=Cartesian  TranslationLengthUnit=mm  TranslationStandardAxis=+Z  TranslationStandardOffset=0  TranslationCartesianOffset=[55.8872 -79.97229999999999 18.7791]  TranslationROffset=0  TranslationROffsetUnits=m  TranslationZOffset=0  TranslationZOffsetUnits=m  TranslationThetaOffset=0  TranslationThetaOffsetUnits=deg  RotationMethod=ArbitraryAxis  RotationAngleUnits=rad  RotationStandardAxis=+Z  RotationAngle=1.6178481128137681  RotationArbitraryAxis=[0.21194708467810197 -0.21194708467810194 0.95402141830930975]  FollAlignAxisA=+X  BaseAlignAxisA=+Y  FollAlignAxisB=+Y  BaseAlignAxisB=+Z  BlockFunction=simmechanics.library.frames_transforms.rigid_transform
  Transform3 : sm_lib/Frames and Transforms/Rigid Transform  TranslationMethod=Cartesian  TranslationLengthUnit=mm  TranslationStandardAxis=+Z  TranslationStandardOffset=0  TranslationCartesianOffset=[111.887 -79.97229999999999 18.7791]  TranslationROffset=0  TranslationROffsetUnits=m  TranslationZOffset=0  TranslationZOffsetUnits=m  TranslationThetaOffset=0  TranslationThetaOffsetUnits=deg  RotationMethod=ArbitraryAxis  RotationAngleUnits=rad  RotationStandardAxis=+Z  RotationAngle=3.1415926535897931  RotationArbitraryAxis=[0 0.36955459314218925 0.92920901991291016]  FollAlignAxisA=+X  BaseAlignAxisA=+Y  FollAlignAxisB=+Y  BaseAlignAxisB=+Z  BlockFunction=simmechanics.library.frames_transforms.rigid_transform
  Transform4 : sm_lib/Frames and Transforms/Rigid Transform  TranslationMethod=Cartesian  TranslationLengthUnit=mm  TranslationStandardAxis=+Z  TranslationStandardOffset=0  TranslationCartesianOffset=[217.98699999999999 -6.5523399999999992 18.7791]  TranslationROffset=0  TranslationROffsetUnits=m  TranslationZOffset=0  TranslationZOffsetUnits=m  TranslationThetaOffset=0  TranslationThetaOffsetUnits=deg  RotationMethod=ArbitraryAxis  RotationAngleUnits=rad  RotationStandardAxis=+Z  RotationAngle=2.0943951023931953  RotationArbitraryAxis=[0.57735026918962584 0.57735026918962584 0.57735026918962584]  FollAlignAxisA=+X  BaseAlignAxisA=+Y  FollAlignAxisB=+Y  BaseAlignAxisB=+Z  BlockFunction=simmechanics.library.frames_transforms.rigid_transform
  Transform5 : sm_lib/Frames and Transforms/Rigid Transform  TranslationMethod=Cartesian  TranslationLengthUnit=mm  TranslationStandardAxis=+Z  TranslationStandardOffset=0  TranslationCartesianOffset=[16.944099999999999 -79.97229999999999 18.7791]  TranslationROffset=0  TranslationROffsetUnits=m  TranslationZOffset=0  TranslationZOffsetUnits=m  TranslationThetaOffset=0  TranslationThetaOffsetUnits=deg  RotationMethod=None  RotationAngleUnits=deg  RotationStandardAxis=+Z  RotationAngle=0  RotationArbitraryAxis=[0 0 1]  FollAlignAxisA=+X  BaseAlignAxisA=+Y  FollAlignAxisB=+Y  BaseAlignAxisB=+Z  BlockFunction=simmechanics.library.frames_transforms.rigid_transform
  x15060_Ecrou_24_Ecrou_Hm_M16_1_RIGID : Subsystem
  x15060_M_01073_Interface_ar_verin_AA_DEFAULT_1_RIGID : Subsystem
  x15060_NLM_Embout_a_rotule_M16_Pas_a_droite_27627_16_1_RIGID : Subsystem
  x15060_Verin_LA36_Course_100_mm_1_RIGID : Subsystem
  F1 : PMIOPort  Port=1  Side=Left
  F : PMIOPort  Port=2  Side=Left
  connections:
  Transform/LConn1 -- ReferenceFrame/RConn1 -- Transform1/LConn1 -- Transform2/LConn1 -- Transform3/LConn1 -- Transform4/LConn1 -- Transform5/LConn1
  Transform/RConn1 -- F/RConn1
  Transform1/RConn1 -- F1/RConn1
  Transform2/RConn1 -- x15060_Ecrou_24_Ecrou_Hm_M16_1_RIGID/LConn1
  Transform3/RConn1 -- x15060_M_01073_Interface_ar_verin_AA_DEFAULT_1_RIGID/LConn1
  Transform4/RConn1 -- x15060_Verin_LA36_Course_100_mm_1_RIGID/LConn1
  Transform5/RConn1 -- x15060_NLM_Embout_a_rotule_M16_Pas_a_droite_27627_16_1_RIGID/LConn1

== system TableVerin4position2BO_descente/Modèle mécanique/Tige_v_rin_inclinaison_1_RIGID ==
  ReferenceFrame : sm_lib/Frames and Transforms/Reference Frame  BlockFunction=simmechanics.library.frames_transforms.reference_frame
  Transform : sm_lib/Frames and Transforms/Rigid Transform  TranslationMethod=Cartesian  TranslationLengthUnit=mm  TranslationStandardAxis=+Z  TranslationStandardOffset=0  TranslationCartesianOffset=[498.38299999999998 -79.97229999999999 18.7791]  TranslationROffset=0  TranslationROffsetUnits=m  TranslationZOffset=0  TranslationZOffsetUnits=m  TranslationThetaOffset=0  TranslationThetaOffsetUnits=deg  RotationMethod=ArbitraryAxis  RotationAngleUnits=deg  RotationStandardAxis=+Z  RotationAngle=-90  RotationArbitraryAxis=[1 0 0]  FollAlignAxisA=+X  BaseAlignAxisA=+Y  FollAlignAxisB=+Y  BaseAlignAxisB=+Z  BlockFunction=simmechanics.library.frames_transforms.rigid_transform
  Transform1 : sm_lib/Frames and Transforms/Rigid Transform  TranslationMethod=Cartesian  TranslationLengthUnit=mm  TranslationStandardAxis=+Z  TranslationStandardOffset=0  TranslationCartesianOffset=[483.03179999999998 -79.97229999999999 18.7791]  TranslationROffset=0  TranslationROffsetUnits=m  TranslationZOffset=0  TranslationZOffsetUnits=m  TranslationThetaOffset=0  TranslationThetaOffsetUnits=deg  RotationMethod=ArbitraryAxis  RotationAngleUnits=rad  RotationStandardAxis=+Z  RotationAngle=2.0943951023931953  RotationArbitraryAxis=[0.57735026918962584 0.57735026918962584 0.57735026918962584]  FollAlignAxisA=+X  BaseAlignAxisA=+Y  FollAlignAxisB=+Y  BaseAlignAxisB=+Z  BlockFunction=simmechanics.library.frames_transforms.rigid_transform
  Transform2 : sm_lib/Frames and Transforms/Rigid Transform  TranslationMethod=Cartesian  TranslationLengthUnit=mm  TranslationStandardAxis=+Z  TranslationStandardOffset=0  TranslationCartesianOffset=[468.38299999999998 -79.97229999999999 18.7791]  TranslationROffset=0  TranslationROffsetUnits=m  TranslationZOffset=0  TranslationZOffsetUnits=m  TranslationThetaOffset=0  TranslationThetaOffsetUnits=deg  RotationMethod=ArbitraryAxis  RotationAngleUnits=rad  RotationStandardAxis=+Z  RotationAngle=1.5707963267948968  RotationArbitraryAxis=[-1 -0 -0]  FollAlignAxisA=+X  BaseAlignAxisA=+Y  FollAlignAxisB=+Y  BaseAlignAxisB=+Z  BlockFunction=simmechanics.library.frames_transforms.rigid_transform
  Transform3 : sm_lib/Frames and Transforms/Rigid Transform  TranslationMethod=Cartesian  TranslationLengthUnit=mm  TranslationStandardAxis=+Z  TranslationStandardOffset=0  TranslationCartesianOffset=[468.38299999999998 -79.97229999999999 18.7791]  TranslationROffset=0  TranslationROffsetUnits=m  TranslationZOffset=0  TranslationZOffsetUnits=m  TranslationThetaOffset=0  TranslationThetaOffsetUnits=deg  RotationMethod=ArbitraryAxis  RotationAngleUnits=rad  RotationStandardAxis=+Z  RotationAngle=3.1415926535897931  RotationArbitraryAxis=[0 -0.69484755531927389 0.71915705855315692]  FollAlignAxisA=+X  BaseAlignAxisA=+Y  FollAlignAxisB=+Y  BaseAlignAxisB=+Z  BlockFunction=simmechanics.library.frames_transforms.rigid_transform
  x15060_Tige_Verin_LA36_AA_DEFAULT_1_RIGID : Subsystem
  x15060_Verin_LA36_Rotule_tige_verin_AA_DEFAULT_1_RIGID : Subsystem
  F : PMIOPort  Port=1  Side=Left
  F1 : PMIOPort  Port=2  Side=Right
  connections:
  Transform/LConn1 -- ReferenceFrame/RConn1 -- Transform2/LConn1 -- Transform3/LConn1 -- Transform1/LConn1
  Transform/RConn1 -- F/RConn1
  Transform1/RConn1 -- F1/RConn1
  Transform2/RConn1 -- x15060_Verin_LA36_Rotule_tige_verin_AA_DEFAULT_1_RIGID/LConn1
  Transform3/RConn1 -- x15060_Tige_Verin_LA36_AA_DEFAULT_1_RIGID/LConn1
